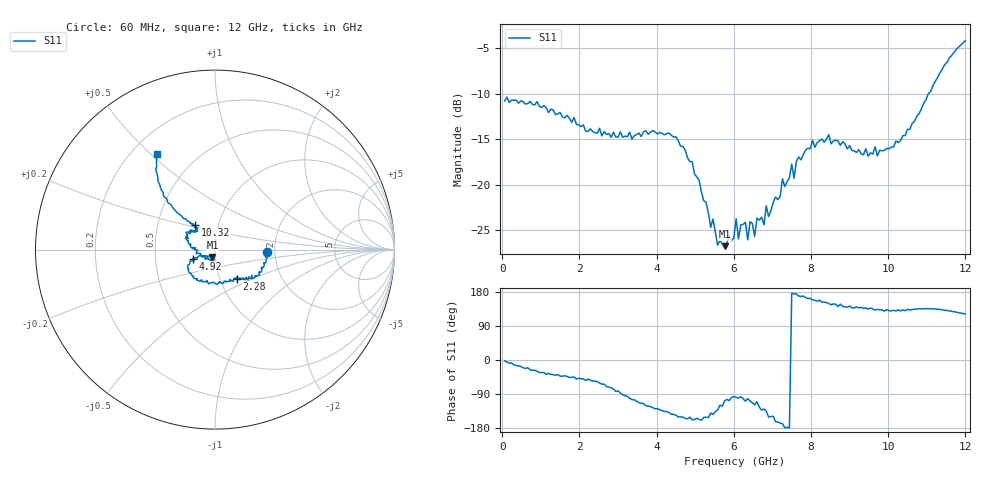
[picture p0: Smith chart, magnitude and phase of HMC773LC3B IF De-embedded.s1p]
! Hittite Microwave Corporation
! 20 Alpha Road
! Chelmsford, MA 01824
! http://www.hittite.com
! Tel: 978-250-3343
! Fax: 978-250-3373
! Device:  HMC773LC3B
! Description: GaAS MMIC Fundamental Mixer
! Frequency:  6-  26 GHz Mixer
! Package:  LC3B - 3x3 mm QFN Ceramic High frequency SMT Package: 12 pin
! Ports
!  Pin  2  = LO
!  Pin  5  = IF
!  pin  8  = RF
! Data:  The device was measured on evaluation board 125040-1.
!  The evaluation circuit board was modeled and simulated.  This was use
!  to removed the evaluation board circuit from the measured data.
!  The reference plane is the center of the package pin.
! Misc:
! Date Measured:  09-10-2009
! Date:  09-10-2009
! Note:
!  Hittite supplies this data as a sample of measured data at the package pin for
!  for this package product.  Your particular data for this product may vary.
!  Data was taken at 25 degrees C.
!  Hittite reserves the right to change this data at anytime.
# MHz S MA R 50
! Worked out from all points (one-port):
!   200 points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, 60 MHz to 12 GHz, reference 50 ohm
!   lowest |S11| = -26.8 dB at 5.76 GHz (marker M1), VSWR 1.10, Z = 48.4 - j4.23 ohm
!   |S11| at or under -10 dB: start of sweep to 11.04 GHz
!   S11 on the Smith chart (normalised r, x): 60 MHz: 1.81, -0.05; 2.28 GHz: 1.20, -0.41; 4.92 GHz: 0.78, -0.08; 10.32 GHz: 0.77, +0.22; 12 GHz: 0.30, +0.52
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60  0.2883 -2.3
1560  0.2356 -42.8
2280  0.2028 -53.1
3060  0.1949 -87.0
4560  0.1747 -150.2
4920  0.1338 -157.9
5400  0.0582 -139.8
5760  0.04586 -107.9
6000  0.05099 -96.7
6060  0.06486 -98.6
6120  0.05024 -100.8
6300  0.06204 -108.6
6360  0.0497 -101.7
6420  0.06257 -108.3
6540  0.05192 -118.3
6600  0.0654 -110.2
6780  0.06016 -129.5
6840  0.07646 -134.9
6900  0.06678 -150.5
7500  0.1297 175.8
7560  0.1083 174.9
7620  0.1346 174.5
8040  0.1753 159.0
9060  0.1541 137.5
10320  0.175 129.5
10560  0.2012 131.9
11100  0.3253 135.4
12000  0.6212 121.3
